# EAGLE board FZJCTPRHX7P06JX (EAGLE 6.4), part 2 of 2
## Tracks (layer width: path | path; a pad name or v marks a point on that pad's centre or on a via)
CLOCK  (via drill 0.6 pad 1.27)
  Top 0.406: v26.16,28.7 26.16,24.64 27.69,23.11 29.46,23.11 38.1,14.48 40.64,14.48 41.27,13.84 IC1.11 | IC21.4 30.25,6.58 29.46,7.37 29.46,17.27 22.86,23.88 v22.86,28.7 22.86,32.51 12.19,43.18 v12.19,50.04 13.46,51.31 15.75,51.31 16.33,50.72 IC3.11 | IC2.11 28.27,32.44 27.43,33.27 v26.16,33.27 | IC4.11 16.33,69.52 14.99,70.87 13.46,70.87 v11.94,69.34 11.94,56.9 v12.19,56.64 | IC6.11 39.8,81.86 v39.62,81.79 40.39,81.79 49.78,72.39 v54.1,72.39 | IC15.11 43.26,89.84 42.93,90.17 40.39,90.17 39.62,89.41 v39.62,86.87 | IC5.11 6.02,89.84 6.86,90.68 6.86,92.71 10.16,96.01 11.94,96.01 | v39.62,92.96 33.27,92.96 29.72,96.52 17.78,96.52 17.27,96.01 11.94,96.01 | IC10.11 73.84,8.71 72.39,10.16 v72.39,13.21 | IC7.11 54.03,63.32 v54.1,63.25 | v54.1,67.31 54.1,68.58 55.12,69.6 56.39,69.6 56.72,69.27 IC14.11 | v54.1,49.28 54.1,50.04 54.86,50.8 56.39,50.8 56.72,50.47 IC13.11 | IC9.11 65.96,25.73 v66.04,25.65 | v66.04,30.23 66.04,31.24 67.31,32.51 69.34,32.51 69.67,32.18 IC12.11 73.84,32.18 75.18,33.53 75.18,35.81 78.49,39.12 88.9,39.12 89.92,38.1 94.23,38.1 95,38.86 95,43.76 | IC8.11 v54.03,45.29 | v54.1,41.15 60.45,34.8 v66.04,34.8 | IC16.11 81.1,82.88 82.55,84.33 85.6,84.33 86.69,83.24 IC17.11 86.69,79.17 94.49,71.37 95,71.37 96.52,69.85 96.52,62.48 96.14,62.1 | IC18.11 93.9,62.05 94.23,61.72 95.76,61.72 96.14,62.1 | IC19.11 95,43.76 | 95,43.76 95.07,43.76 97.28,45.97 97.28,60.96 96.14,62.1 | v11.94,95.25 11.94,96.01 | IC11.11 80.09,14.4 v79.5,14.99
  Bottom 0.406: v26.16,33.27 v26.16,28.7 v22.86,28.7 | v12.19,56.64 v12.19,50.04 | v39.62,81.79 v39.62,86.87 v39.62,92.96 | v54.1,72.39 v54.1,67.31 v54.1,63.25 v54.1,49.28 54.03,49.2 v54.03,45.29 54.03,41.22 v54.1,41.15 | v66.04,34.8 v66.04,30.23 v66.04,25.65 66.04,19.56 v72.39,13.21 74.17,14.99 v79.5,14.99 | v11.94,69.34 v11.94,95.25
CLOCK2  (via drill 0.6)  (2 unrouted)
  Top 0.305: IC20.17 180.34,8.89 179.2,10.03 IC22.11 179.2,15.11 v180.34,16.26 | v192.02,16.76 192.15,16.64 IC23.11 | IC24.11 181.23,33.4 v181.1,33.53
  Bottom 0.305: v180.34,16.26 v192.02,16.76
D8
  Top 0.406: U$1.11 7.37,5.84 11.68,1.52 20.57,1.52 21.34,2.29 21.34,4.06 22.58,5.31 IC21.18
D11
  Top 0.406: U$1.14 19.53,6.58 IC21.17
D13
  Top 0.406: U$1.16 20.32,10.92 21.34,9.91 21.34,8.89 22.38,7.85 IC21.16
DATA
  Top 0.406: IC21.3 35.28,5.31 40.01,10.03 IC1.14
DATA2  (1 unrouted)
  Top 0.305: IC20.15 183.67,11.4 183.01,12.06 IC22.14
GND  (via drill 0.6, 0.6 pad 1.27)  (3 unrouted)
  Top 0.305: v179.32,5.59 179.43,5.7 IC20.21 188.36,5.7 188.47,5.59 | 188.47,5.59 188.47,5.08 188.65,4.9 IC20.3 191.59,4.9 192.02,5.33 | 188.47,5.59 188.47,6.35 188.61,6.5 IC20.5 | IC24.13 185.55,30.86 186.94,32.26 186.94,35.31 187.58,35.94 IC24.8 190.63,35.94 191.52,35.05 193.29,35.05 194.69,33.66 U$52.- | IC23.13 194.69,17.02 193.93,17.78 189.99,17.78 189.61,18.16 IC23.8 | U$53.- 193.55,10.16 192.53,9.14 192.53,5.84 192.02,5.33 | U$75.1 S1.P$1 174.9,22.96 176.66,21.21 IC22.8 176.66,17.65 v177.04,17.27 | v181.61,17.27 181.74,17.14 IC22.13 181.74,12.06 v181.86,11.94 | U$63.1 192.26,5.1 192.02,5.33
  Top 0.406: 38.99,11.56 39.24,11.3 IC1.13 46.1,11.3 46.99,12.19 46.99,15.75 47.62,16.38 IC1.8 49.02,16.41 v49.02,18.03 | 38.99,11.56 36.35,14.2 | 36.35,14.2 28.96,21.59 27.18,21.59 24.64,24.13 24.64,29.46 25.15,29.97 | IC21.10 36.35,14.2 | 25.15,29.97 25.4,30.23 27.69,30.23 28.02,29.9 IC2.13 33.45,29.9 34.04,30.48 34.04,34.29 34.72,34.98 IC2.8 | IC3.8 22.78,53.26 22.1,52.58 22.1,49.02 21.26,48.18 IC3.13 15.67,48.18 v15.24,47.75 | IC5.8 8.56,92.38 7.87,91.69 7.87,88.14 7.04,87.3 IC5.13 1.6,87.3 v1.52,87.38 | IC15.8 49.2,92.38 48.51,91.69 48.51,88.14 47.68,87.3 IC15.13 42.85,87.3 39.95,84.4 IC6.13 35.13,84.4 33.53,82.8 33.53,80.01 32.84,79.32 IC6.8 30.48,79.32 | J1.2 6.6,73.91 v1.52,78.99 | v15.24,67.06 15.32,66.98 IC4.13 20.75,66.98 21.84,68.07 21.84,71.63 22.28,72.06 IC4.8 24.56,72.06 v25.15,72.64 | IC11.8 86.54,16.94 85.85,16.26 85.85,13.72 84,11.86 IC11.13 79.93,11.86 79.32,11.25 v78.23,11.25 | IC13.8 62.66,53.01 61.47,51.82 61.47,49.53 59.87,47.93 IC13.13 57.96,47.83 IC8.13 49.61,47.83 v49.02,47.24 48.77,46.99 48.77,44.2 47.32,42.75 IC8.8 | 47.07,60.78 48.26,61.98 48.26,64.77 49.35,65.86 IC7.13 54.69,65.86 55.55,66.73 IC14.13 59.87,66.73 61.47,68.33 61.47,70.87 62.41,71.81 IC14.8 64.11,73.05 v63.5,73.66 | 47.07,60.78 IC7.8 | IC18.13 90.75,64.59 89.15,62.99 89.15,60.2 88.47,59.51 88.39,59.51 | 88.39,59.51 IC18.8 | IC19.13 90.75,46.3 89.28,44.83 | 89.28,44.83 88.9,44.45 88.9,41.91 88.21,41.22 IC19.8 84.51,41.22 v84.33,41.4 v75.69,41.4 | 47.07,60.78 47.07,56.31 v49.02,54.36 | IC17.8 82.6,87.43 80.59,85.42 IC16.13 77.04,85.42 75.69,84.07 75.69,82.04 73.99,80.34 IC16.8 72.49,79.91 74.68,77.72
  Top 0.406: IC17.13 89.23,79.93 91.19,77.98 v91.69,77.98 | v80.01,77.98 79.76,77.72 74.68,77.72 | v71.37,77.47 71.63,77.72 74.68,77.72 | v79.25,36.32 78.28,35.36 IC12.8 | v56.13,21.59 57.56,23.01 IC9.8 59.26,23.19 60.71,24.64 60.71,26.92 62.05,28.27 IC9.13 66.37,28.27 67.74,29.64 IC12.13 75.62,29.64 v75.69,29.72 75.69,27.43 76.2,26.92 76.2,24.89 77.22,23.88 v77.47,23.88 | 30.3,79.32 30.48,79.32 | v25.15,75.69 26.85,75.69 30.48,79.32 | IC21.19 28.47,4.04 29.74,2.77 IC21.1 36.8,2.77 v37.59,3.56 | U$1.23 19.3,28.7 v21.34,30.73 | v24.38,30.73 25.15,29.97 | v89.15,45.47 89.28,44.83 | v89.15,55.63 88.39,56.39 88.39,59.51 | IC10.13 v78.23,11.25 | v77.72,16.76 78.23,16.26 v78.23,11.25 | v71.37,4.32 70.1,5.59 IC10.8 | v37.59,9.91 37.59,10.16 38.99,11.56 | U$53.- IC23.13
  Top 0.61: U$1.4 2.29,23.62 1.52,24.38 1.52,35.81 6.6,40.89 | J4.2 6.6,40.89 | C1.- 10.67,36.83 6.6,40.89
  Top 0.813: J4.2 v6.6,47.75 J3.2 J2.2 v6.6,67.06 J1.2 | U$1.4 7.62,23.62 12.7,28.7 U$1.23
  Bottom 0.305: v179.32,5.59 179.32,9.4 v181.86,11.94 | U$52.- U$53.- | v177.04,17.27 v181.61,17.27
  Bottom 0.406: v6.6,47.75 v15.24,47.75 | v1.52,78.99 v1.52,87.38 | v15.24,67.06 v6.6,67.06 | v49.02,54.36 v49.02,47.24 | v91.69,77.98 v80.01,77.98 | v63.5,73.66 67.31,77.47 v71.37,77.47 | v79.25,36.32 v84.33,41.4 | v49.02,18.03 52.58,21.59 v56.13,21.59 | v25.15,72.64 v25.15,75.69 | v21.34,30.73 v24.38,30.73 | v89.15,55.63 v89.15,45.47 | v75.69,29.72 v75.69,41.4 | v77.47,23.88 77.72,23.62 v77.72,16.76 | v78.23,11.25 71.37,4.39 v71.37,4.32 | v37.59,3.56 v37.59,9.91
  pour Top (isolate 0.61): 0.76,99.31 99.06,99.31 99.06,1.02 99.06,0.76 0.76,0.76
LATCH  (via drill 0.6 pad 1.27)  (2 unrouted)
  Top 0.406: IC2.12 27.76,31.17 27.43,31.5 25.65,31.5 13.72,43.43 13.72,49.02 v14.48,49.78 15.75,49.78 16.08,49.45 IC3.12 | IC4.12 16.08,68.25 15.75,68.58 14.73,68.58 v14.22,69.09 13.46,68.33 13.46,57.4 v14.48,56.39 | IC15.12 41.33,88.57 v41.15,88.39 | IC5.12 2.36,88.57 1.52,89.41 1.52,94.49 5.59,98.55 v14.22,98.55 33.53,98.55 37.34,94.74 v41.15,94.74 | IC7.12 55.7,64.59 v55.88,64.77 | v55.88,68.07 55.96,68 IC14.12 | IC10.12 74.6,9.98 73.91,10.67 v73.91,11.68 | v55.88,73.41 55.37,73.91 49.78,73.91 41.15,82.55 v41.15,83.31 40.97,83.13 IC6.12 | IC8.12 55.8,46.56 v55.88,46.48 | v55.88,49.28 57.99,49.28 IC13.12 | v68.33,30.99 68.4,30.91 IC12.12 74.35,30.91 76.2,32.77 76.2,35.31 78.99,38.1 88.39,38.1 90.68,35.81 v95.5,35.81 | IC9.12 67.39,27 v68.33,27.94 | v55.88,41.91 61.47,36.32 67.06,36.32 68.07,35.31 v68.33,35.31 | IC16.12 80.85,84.15 82.04,85.34 86.36,85.34 87.96,83.74 IC17.12 87.96,79.68 95,72.64 95.76,72.64 98.3,70.1 v98.3,63.25 | v94.74,63.25 94.67,63.32 IC18.12 | IC19.12 94.56,45.03 95.89,46.35 | 95.89,46.35 96.01,46.48 96.01,54.86 v94.74,56.13 | v95.5,46.74 95.89,46.35 | IC1.12 40.01,12.57 v39.88,12.7 | IC11.12 79.58,13.13 v79.5,13.21 | IC21.2 36.04,4.04 37.34,5.33 38.61,5.33 v39.88,6.6
  Bottom 0.406: v14.48,56.39 v14.48,49.78 | v41.15,83.31 v41.15,88.39 v41.15,94.74 | v55.88,73.41 v55.88,68.07 v55.88,64.77 v55.88,49.28 v55.88,46.48 v55.88,41.91 | v68.33,27.94 v68.33,30.99 v68.33,35.31 | v98.3,63.25 v94.74,63.25 v94.74,56.13 | v95.5,35.81 v95.5,46.74 | v14.22,69.09 v14.22,98.55 | v39.88,12.7 v39.88,6.6 | v73.91,11.68 75.44,13.21 v79.5,13.21
LATCH2  (via drill 0.6)  (1 unrouted)
  Top 0.254: 180.47,11.3 183.13,8.64
  Top 0.305: IC23.12 193.42,12.32 192.79,11.68 184.91,11.68 184.47,11.25 IC20.14 184.47,8.96 184.15,8.64 183.13,8.64 | IC22.12 180.47,11.3 | IC24.12 181.23,32.13 v181.1,32
MISO  (1 unrouted)
N$1  (1 unrouted)
  Top 0.61: U$1.5 2.29,21.08
  Top 0.813: R160.1 113.26,99.97 U$55.1
N$2
  Top 0.61: 100.08,10.16 161.04,10.16 | 100.08,20.32 161.04,20.32 | 100.08,30.48 161.04,30.48 | 100.08,40.64 161.04,40.64 | 100.08,50.8 161.04,50.8 | 100.08,60.96 161.04,60.96 | 100.08,71.12 161.04,71.12 | 100.08,81.28 161.04,81.28 | 100.08,0 110.24,0 | 110.24,0 120.4,0 | 120.4,0 130.56,0 | 130.56,0 140.72,0 | 140.72,0 150.88,0 | 100.08,91.44 110.24,91.44 | 110.24,91.44 120.4,91.44 | 120.4,91.44 130.56,91.44 | 130.56,91.44 140.72,91.44 | 140.72,91.44 150.88,91.44 | 150.88,91.44 161.04,91.44 161.04,81.28 | 110.24,0 110.24,91.44 | 120.4,0 120.4,91.44 | 130.56,0 130.56,91.44 | 140.72,0 140.72,91.44 | 150.88,0 150.88,91.44 | 161.04,10.16 161.04,0 150.88,0 | 161.04,10.16 161.04,20.32 | 161.04,20.32 161.04,30.48 | 161.04,30.48 161.04,40.64 | 161.04,40.64 161.04,50.8 | 161.04,50.8 161.04,60.96 | 161.04,60.96 161.04,71.12 | 161.04,71.12 161.04,81.28 | 100.08,91.44 100.08,100.08 0,100.08 0,0 100.08,0 | 100.08,91.44 100.08,0
N$3  (via drill 0.6 pad 1.78)
  other vias: 2.29,21.08
N$4
  Top 0.305: IC22.15 184.28,14.86 185.74,16.32 R168.1
N$5
  Top 0.406: R81.2 74.67,2.75 U$28.1
N$6  (via drill 0.6 pad 1.27)
  Top 0.406: IC10.9 78.92,6.17 v79.25,5.84 | v79.25,9.14 79.25,9.65 80.19,10.59 IC11.14
  Bottom 0.406: v79.25,5.84 v79.25,9.14
N$7
  Top 0.305: IC22.1 187.71,21.74 R151.1
N$8
  Top 0.305: IC22.2 184.28,21.53 R152.1
N$9
  Top 0.305: R168.2 U$54.1
N$10
  Top 0.305: R151.2 U$56.1
N$11
  Top 0.305: R152.2 U$57.1
N$12
  Top 0.305: R169.2 U$58.1
N$13
  Top 0.305: R153.2 U$59.1
N$14
  Top 0.305: R154.2 U$60.1
N$15
  Top 0.305: U$61.1 173.04,12.89 R170.2
N$16
  Top 0.305: U$62.1 173.04,20.64 R155.2
N$17
  Top 0.305: IC22.3 183.01,22.29 R169.1
N$18
  Top 0.305: IC22.4 181.74,20.95 180.85,21.84 180.85,22.67 R153.1
N$19
  Top 0.305: IC22.5 180.47,20.95 179.83,21.59 179.14,21.59 R154.1
N$20
  Top 0.305: R170.1 175.45,15.24 178.05,15.24 179.2,16.38 IC22.6
N$21
  Top 0.305: IC22.7 177.93,18.67 178.31,18.29 178.31,16.76 177.55,16 176.28,16 174.94,17.34 R155.1
N$22
  Top 0.305: IC23.15 197.23,11.81 197.87,11.18 198.82,11.18 R156.1
N$23  (1 unrouted)
N$24
  Top 0.305: R171.2 202.95,18.1 U$66.1
N$25
  Top 0.305: R157.2 202.44,15.17 U$67.1
N$26
  Top 0.305: R158.2 202.69,21.66 U$68.1
N$27  (1 unrouted)
N$28  (1 unrouted)
N$29
  Top 0.406: IC1.15 45.59,8.76 46.99,7.37 46.99,6.1 50.77,2.31 R1.1
N$30
  Top 0.406: IC1.1 51.97,4.57 R2.1
N$31
  Top 0.406: IC1.2 50.67,8.76 52.6,6.83 R3.1
N$32
  Top 0.406: R1.2 58.41,2.31 U$2.3
N$33
  Top 0.406: R2.2 U$2.2
N$34
  Top 0.406: R3.2 58.41,6.83 U$2.1
N$35
  Top 0.406: R4.2 58.36,9.12 U$3.3
N$36
  Top 0.406: R5.2 58.6,11.35 U$3.2
N$37
  Top 0.406: R6.2 58.52,13.59 U$3.1
N$38
  Top 0.406: R7.2 58.31,15.93 U$4.3
N$39
  Top 0.406: R8.2 58.6,18.36 U$4.2
N$40
  Top 0.406: IC1.3 52.44,10.03 R4.1
N$41
  Top 0.406: IC1.4 54.27,11.3 R5.1
N$42
  Top 0.406: IC1.5 51.94,12.57 52.96,13.59 R6.1
N$43
  Top 0.406: IC1.6 51.27,13.84 R7.1
N$44
  Top 0.406: IC1.7 50.67,15.11 51.56,16 51.56,17.53 52.4,18.36 R8.1
N$45
  Top 0.406: R9.1 37.31,20.6 34.04,23.88 34.04,26.16 32.84,27.36 IC2.15
N$46
  Top 0.406: R9.2 43.8,20.07 58.45,20.07 U$4.1
N$47
  Top 0.406: R10.2 45.08,22.99 U$5.3
N$48
  Top 0.406: R11.2 45.47,25.38 U$5.2
N$49
  Top 0.406: R12.2 45.43,27.61 U$5.1
N$50
  Top 0.406: R13.2 45.26,29.79 U$6.3
N$51
  Top 0.406: R14.2 45.49,32.13 U$6.2
N$52
  Top 0.406: R15.2 45.26,34.37 U$6.1
N$53
  Top 0.406: R16.2 34.73,37.31 U$7.3
N$54
  Top 0.406: R17.2 33.78,39.14 U$7.2
N$55
  Top 0.406: R18.2 34.02,41.38 U$7.1
N$56
  Top 0.406: R19.2 33.17,43.66 U$8.3
N$57
  Top 0.406: R20.2 33.2,45.9 U$8.2
N$58
  Top 0.406: R21.2 32.96,48.13 U$8.1
N$59
  Top 0.406: R22.2 32.84,50.47 U$9.3
N$60
  Top 0.406: R23.2 U$9.2
N$61
  Top 0.406: R24.2 33.04,55.14 U$9.1
N$62
  Top 0.406: R25.2 33.01,57.53 U$10.3
N$63
  Top 0.406: R26.2 33.1,59.92 U$10.2
N$64
  Top 0.406: R27.2 32.86,62.15 U$10.1
N$65
  Top 0.406: R28.2 32.94,64.59 U$11.3
N$66
  Top 0.406: R29.2 33.17,66.93 U$11.2
N$67
  Top 0.406: R30.2 32.94,69.16 U$11.1
N$68
  Top 0.406: U$12.3 33.28,71.4 R31.2
N$69
  Top 0.406: U$12.2 32.99,73.69 R32.2
N$70  (via drill 0.6 pad 1.27)
  Top 0.406: R33.2 18.35,76.96 v21.84,76.96 | v33.53,76.96 33.53,75.15 U$12.1
  Bottom 0.406: v21.84,76.96 v33.53,76.96
N$71
  Top 0.406: R34.2 19.07,80.49 U$13.3
N$72
  Top 0.406: R35.2 19.1,82.73 U$13.2
N$73
  Top 0.406: R36.2 18.87,84.96 U$13.1
N$74
  Top 0.406: R37.2 18.99,87.3 U$14.3
N$75
  Top 0.406: R38.2 U$14.2
N$76
  Top 0.406: R39.2 19.2,91.97 U$14.1
N$77
  Top 0.406: U$15.3 16.67,94.89 R40.2
N$78
  Top 0.406: R41.2 22.61,93.5 U$15.2
N$79
  Top 0.406: R42.2 22.37,91.26 U$15.1
N$80
  Top 0.406: R43.2 22.31,89.08 U$16.3
N$81
  Top 0.406: R44.2 22.07,86.74 U$16.2
N$82
  Top 0.406: R45.2 22.31,84.51 U$16.1
N$83
  Top 0.406: U$17.3 22.73,82.27 R46.2
N$84
  Top 0.406: R47.2 23.08,80.95 U$17.2
N$85
  Top 0.406: U$17.1 23.25,77.75 R48.2
N$86
  Top 0.406: R49.2 36.18,74.95 U$18.3
N$87
  Top 0.406: R50.2 36.14,72.72 U$18.2
N$88
  Top 0.406: R51.2 36.38,70.48 U$18.1
N$89
  Top 0.406: R52.2 36.25,68.15 U$19.3
N$90
  Top 0.406: R53.2 U$19.2
N$91
  Top 0.406: R54.2 36.3,63.73 U$19.1
N$92
  Top 0.406: R55.2 36.58,61.59 U$20.3
N$93
  Top 0.406: R56.2 36.2,59.21 U$20.2
N$94
  Top 0.406: R57.2 36.48,56.72 U$20.1
N$95
  Top 0.406: R58.2 36.41,54.53 U$21.3
N$96
  Top 0.406: R59.2 36.17,52.2 U$21.2
N$97
  Top 0.406: R60.2 36.41,49.96 U$21.1
N$98
  Top 0.406: R61.2 36.48,47.73 U$22.3
N$99
  Top 0.406: R62.2 36.2,45.44 U$22.2
N$100
  Top 0.406: R63.2 36.33,43.2 U$22.1
N$101
  Top 0.406: R64.2 47.83,38.98 U$23.3
N$102
  Top 0.406: R65.2 48.26,37.41 U$23.2
N$103
  Top 0.406: R66.2 48.19,35.18 U$23.1
N$104
  Top 0.406: R67.2 48.32,32.84 U$24.3
N$105
  Top 0.406: R68.2 U$24.2
N$106
  Top 0.406: R69.2 48.37,28.42 U$24.1
N$107
  Top 0.406: R70.2 48.39,26.04 U$25.3
N$108
  Top 0.406: R71.2 48.26,23.9 U$25.2
N$109
  Top 0.406: R72.2 48.29,21.67 U$25.1
N$110
  Top 0.406: R73.2 61.42,20.5 U$26.3
N$111
  Top 0.406: R74.2 61.19,18.16 U$26.2
N$112
  Top 0.406: R75.2 61.42,15.93 U$26.1
N$113
  Top 0.406: R76.2 61.5,13.69 U$27.3
N$114
  Top 0.406: R77.2 61.21,11.4 U$27.2
N$115
  Top 0.406: R78.2 61.35,9.17 U$27.1
N$116
  Top 0.406: R79.2 61.32,6.88 U$28.3
N$117
  Top 0.406: R80.2 61.29,4.65 U$28.2
N$118
  Top 0.406: R82.2 97.1,5 U$29.3
N$119
  Top 0.406: R83.2 U$29.2
N$120
  Top 0.406: R84.2 97.05,9.42 U$29.1
N$121
  Top 0.406: R85.2 97.02,11.81 U$30.3
N$122
  Top 0.406: R86.2 97.1,14.2 U$30.2
N$123
  Top 0.406: R87.2 96.87,16.43 U$30.1
N$124
  Top 0.406: R88.2 90.05,20.71 88.75,19.41 U$31.3
N$125
  Top 0.406: R89.2 85.81,20.83 87.25,20.83 U$31.2
N$126
  Top 0.406: R90.2 87.1,22.68 U$31.1
N$127
  Top 0.406: R91.2 87.47,25.17 U$32.3
N$128
  Top 0.406: R92.2 87.76,27.46 U$32.2
N$129
  Top 0.406: R93.2 87.62,29.69 U$32.1
N$130
  Top 0.406: R94.2 87.65,31.98 U$33.3
N$131
  Top 0.406: R95.2 87.68,34.21 U$33.2
N$132
  Top 0.406: R96.2 87.45,36.45 U$33.1
N$133
  Top 0.406: R97.2 73.6,38.79 U$34.3
N$134
  Top 0.406: R98.2 U$34.2
N$135
  Top 0.406: R99.2 73.55,43.2 U$34.1
N$136
  Top 0.406: R100.2 73.27,45.59 U$35.3
N$137
  Top 0.406: R101.2 73.66,47.98 U$35.2
N$138
  Top 0.406: R102.2 73.63,50.22 U$35.1
N$139
  Top 0.406: R103.2 73.45,52.65 U$36.3
N$140
  Top 0.406: R104.2 73.69,54.99 U$36.2
N$141
  Top 0.406: R105.2 72.94,57.73 U$36.1
N$142
  Top 0.406: R106.2 73.37,59.97 U$37.3
N$143
  Top 0.406: R107.2 73.66,62.26 U$37.2
N$144
  Top 0.406: R108.2 73.53,64.49 U$37.1
N$145
  Top 0.406: R109.2 73.55,66.78 U$38.3
N$146
  Top 0.406: R110.2 73.58,69.01 U$38.2
N$147
  Top 0.406: R111.2 73.35,71.25 U$38.1
N$148
  Top 0.406: R112.2 65.22,75.18 61.07,75.18 U$39.3
N$149
  Top 0.406: R113.2 U$39.2
N$150
  Top 0.406: R114.2 59.96,80.29 U$39.1
N$151
  Top 0.406: R115.2 59.94,82.68 U$40.3
N$152
  Top 0.406: R116.2 60.02,85.06 U$40.2
N$153
  Top 0.406: R117.2 59.78,87.3 U$40.1
N$154
  Top 0.406: R118.2 59.86,89.74 U$41.3
N$155
  Top 0.406: R119.2 60.1,92.08 U$41.2
N$156
  Top 0.406: R120.2 59.86,94.31 U$41.1
N$157
  Top 0.406: R121.2 63.15,94.46 U$42.3
N$158
  Top 0.406: R122.2 62.87,92.18 U$42.2
N$159
  Top 0.406: R123.2 63,89.94 U$42.1
N$160
  Top 0.406: R124.2 62.97,87.66 U$43.3
N$161
  Top 0.406: R125.2 62.94,85.42 U$43.2
N$162
  Top 0.406: R126.2 63.18,83.19 U$43.1
N$163
  Top 0.406: R127.2 63.05,80.85 U$44.3
N$164
  Top 0.406: R128.2 U$44.2
N$165  (via drill 0.6 pad 1.27)
  Top 0.406: R129.2 94.17,76.71 96.01,76.71 v96.27,76.45 | 82.59,76.66 v82.8,76.45 82.55,76.71 74.68,76.71 73.91,75.95 69.85,75.95 69.13,76.66 U$44.1
  Bottom 0.406: v82.8,76.45 v96.27,76.45
N$166
  Top 0.406: R130.2 96.14,96.39 U$45.3
N$167
  Top 0.406: R131.2 93.75,96.77 U$45.2
N$168
  Top 0.406: R132.2 91.52,96.74 U$45.1
N$169
  Top 0.406: R133.2 89.33,96.56 U$46.3
N$170
  Top 0.406: R134.2 87,96.8 U$46.2
N$171
  Top 0.406: R135.2 84.76,96.56 U$46.1
N$172  (via drill 0.6 pad 1.27)
  Top 0.406: v81.28,96.77 82.53,95.53 R136.2
  Bottom 0.406: U$47.3 76.91,92.41 v76.96,92.46 v81.28,96.77
N$173
  Top 0.406: R137.2 77.47,73.64 U$47.2
N$174
  Top 0.406: R138.2 77.23,71.4 U$47.1
N$175
  Top 0.406: R139.2 77.07,69.11 U$48.3
N$176
  Top 0.406: R140.2 77.04,66.88 U$48.2
N$177
  Top 0.406: R141.2 77.27,64.64 U$48.1
N$178
  Top 0.406: R142.2 77.4,62.31 U$49.3
N$179
  Top 0.406: R143.2 U$49.2
N$180
  Top 0.406: R144.2 77.2,57.63 U$49.1
N$181
  Top 0.406: R145.2 77.48,54.48 U$50.3
N$182
  Top 0.406: R146.2 77.09,52.09 U$50.2
N$183
  Top 0.406: R147.2 77.12,49.86 U$50.1
N$184
  Top 0.406: R148.2 77.3,47.68 U$51.3
N$185
  Top 0.406: R149.2 77.11,45.49 U$51.2
N$186
  Top 0.406: R150.2 77.25,43.16 U$51.1
N$187  (1 unrouted)
N$188
  Top 0.305: R173.2 U$72.1
N$189
  Top 0.305: R162.2 U$73.1
N$190  (1 unrouted)
N$191
  Top 0.66: 24.89,14.22 27.18,14.22
N$192
  Top 0.66: 24.89,12.95 27.18,12.95
N$193
  Top 0.66: 24.64,11.68 27.18,11.68
N$194
  Top 0.66: 24.64,10.41 27.18,10.41
N$195
  Top 0.66: 24.89,9.14 27.18,9.14
N$196
  Top 0.406: R81.1 83.69,3.17 86.36,5.84 86.36,7.62 84.66,9.32 IC11.15
N$197
  Top 0.406: IC11.1 90.83,5 R82.1
N$198
  Top 0.406: IC11.2 89.74,9.32 91.87,7.19 R83.1
N$199
  Top 0.406: IC11.3 90.25,10.59 91.42,9.42 R84.1
N$200
  Top 0.406: IC11.4 91.91,11.86 R85.1
N$201
  Top 0.406: IC11.5 90.6,13.13 91.67,14.2 R86.1
N$202
  Top 0.406: IC11.6 90.09,14.4 92.13,16.43 R87.1
N$203
  Top 0.406: IC11.7 89.33,15.67 90.86,17.2 R88.1
N$204
  Top 0.406: IC12.15 73.99,27.1 74.68,26.42 74.68,24.64 77.47,21.84 80.26,21.84 81.66,20.45 R89.1
N$205
  Top 0.406: IC12.1 81.43,22.68 R90.1
N$206
  Top 0.406: IC12.2 80.64,27.1 R91.1
N$207
  Top 0.406: IC12.3 81.36,28.37 82.27,27.46 R92.1
N$208
  Top 0.406: IC12.4 83.48,29.64 R93.1
N$209
  Top 0.406: IC12.5 81.5,30.91 R94.1
N$210
  Top 0.406: IC12.6 79.93,32.18 81.97,34.21 R95.1
N$211
  Top 0.406: IC12.7 79.68,33.45 82.68,36.45 R96.1
N$212
  Top 0.406: IC13.15 61.04,45.39 61.98,44.45 61.98,41.91 65.1,38.79 R97.1
N$213
  Top 0.406: IC13.1 67.36,40.97 R98.1
N$214
  Top 0.406: IC13.2 65.86,45.39 68.05,43.2 R99.1
N$215
  Top 0.406: IC13.3 67.53,46.66 R100.1
N$216
  Top 0.406: IC13.4 69.51,47.93 R101.1
N$217
  Top 0.406: IC13.5 67.74,49.2 68.76,50.22 R102.1
N$218
  Top 0.406: IC13.6 66.41,50.47 R103.1
N$219
  Top 0.406: IC13.7 65.71,51.74 66.55,52.58 66.55,53.59 67.94,54.99 R104.1
N$220
  Top 0.406: IC14.15 60.27,64.19 61.98,62.48 61.98,60.96 65.2,57.73 R105.1
N$221
  Top 0.406: IC14.1 67.06,59.97 R106.1
N$222
  Top 0.406: IC14.2 66.37,64.19 68.3,62.26 R107.1
N$223
  Top 0.406: IC14.3 66.88,65.46 67.84,64.49 R108.1
N$224
  Top 0.406: IC14.4 68.54,66.73 R109.1
N$225
  Top 0.406: IC14.5 67.23,68 68.25,69.01 R110.1
N$226
  Top 0.406: IC14.6 66.73,69.27 68.71,71.25 R111.1
N$227
  Top 0.406: IC14.7 65.46,70.54 68.06,73.14 R112.1
N$228
  Top 0.406: IC15.15 47.57,84.76 48.51,83.82 48.51,81.79 52.25,78.05 R113.1
N$229
  Top 0.406: IC15.1 53.75,80.29 R114.1
N$230
  Top 0.406: IC15.2 52.4,84.76 54.48,82.68 R115.1
N$231
  Top 0.406: IC15.3 53.42,86.03 54.38,85.06 R116.1
N$232
  Top 0.406: IC15.4 R117.1
N$233
  Top 0.406: IC15.5 52.76,88.57 53.92,89.74 R118.1
N$234
  Top 0.406: IC15.6 52.25,89.84 54.48,92.08 R119.1
N$235
  Top 0.406: IC15.7 51.74,91.11 53.34,92.71 53.34,93.47 54.18,94.31 R120.1
N$236
  Top 0.406: IC16.15 75.87,87.96 74.68,89.15 74.68,89.66 73.91,90.42 73.91,92.46 71.91,94.46 R121.1
N$237
  Top 0.406: IC16.1 69.55,92.18 R122.1
N$238
  Top 0.406: IC16.2 70.79,87.96 68.81,89.94 R123.1
N$239
  Top 0.406: IC16.3 69.02,86.69 R124.1
N$240
  Top 0.406: IC16.4 R125.1
N$241
  Top 0.406: IC16.5 69.67,84.15 68.71,83.19 R126.1
N$242
  Top 0.406: IC16.6 70.43,82.88 68.4,80.85 R127.1
N$243
  Top 0.406: IC16.7 70.94,81.61 69.85,80.52 69.85,79.5 69.01,78.66 R128.1
N$244
  Top 0.406: IC17.15 91.77,79.93 92.93,78.78 R129.1
N$245
  Top 0.406: IC17.1 96.14,90.53 R130.1
N$246
  Top 0.406: IC17.2 91.77,89.23 93.75,91.21 R131.1
N$247
  Top 0.406: IC17.3 90.5,89.74 91.52,90.75 R132.1
N$248
  Top 0.406: IC17.4 89.23,91.61 R133.1
N$249
  Top 0.406: IC17.5 87.96,89.84 87,90.81 R134.1
N$250
  Top 0.406: IC17.6 86.69,89.59 84.76,91.52 R135.1
N$251
  Top 0.406: IC17.7 85.42,89.08 82.79,91.71 R136.1
N$252
  Top 0.406: IC18.15 90.86,67.13 88.65,69.34 88.65,71.37 86.39,73.64 R137.1
N$253
  Top 0.406: IC18.1 83.67,71.4 R138.1
N$254
  Top 0.406: IC18.2 84.26,67.13 R139.1
N$255
  Top 0.406: IC18.3 83.49,65.86 82.47,66.88 R140.1
N$256
  Top 0.406: IC18.4 81.37,64.59 R141.1
N$257
  Top 0.406: IC18.5 83.3,63.32 R142.1
N$258
  Top 0.406: IC18.6 84.91,62.05 82.73,59.87 R143.1
N$259
  Top 0.406: IC18.7 85.42,60.78 82.27,57.63 R144.1
N$260
  Top 0.406: IC19.15 90.86,48.84 88.65,51.05 88.65,52.58 86.74,54.48 R145.1
N$261
  Top 0.406: IC19.1 84.53,52.09 R146.1
N$262
  Top 0.406: IC19.2 84.51,48.84 83.49,49.86 R147.1
N$263
  Top 0.406: IC19.3 82.38,47.57 R148.1
N$264
  Top 0.406: IC19.4 84.4,46.3 83.57,45.47 81.29,45.47 R149.1
N$265
  Top 0.406: IC19.5 84.91,45.03 83.03,43.16 R150.1
N$266
  Top 0.66: 24.89,7.87 27.18,7.87
N$267
  Top 0.66: 24.89,6.6 27.18,6.6
N$268
  Top 0.66: 24.89,5.33 27.18,5.33
N$269
  Top 0.66: 24.89,4.06 27.18,4.06
N$270
  Top 0.66: 24.89,2.79 27.18,2.79
N$271
  Top 0.66: 34.04,14.22 31.5,14.22
N$272
  Top 0.66: 33.78,12.95 31.5,12.95
N$273
  Top 0.305: IC24.1 190.88,27.05 192.53,28.7 R163.1
N$274
  Top 0.305: R162.1 180.15,28.7 181.1,28.7 181.48,28.32 IC24.15
N$275
  Top 0.305: IC23.7 190.88,21.53 R173.1
N$276
  Top 0.406: IC10.7 68.66,7.44 68.07,6.86 68.07,5.33 67.39,4.65 R80.1
N$277
  Top 0.406: IC10.6 68.11,8.71 R79.1
N$278
  Top 0.406: IC10.5 67.13,9.98 66.32,9.17 R78.1
N$279
  Top 0.406: IC10.4 65.47,11.25 R77.1
N$280
  Top 0.406: IC10.3 67.45,12.52 R76.1
N$281
  Top 0.406: R75.1 66.88,15.93 69.01,13.79 IC10.2
N$282
  Top 0.406: IC10.1 67.26,18.16 R74.1
N$283
  Top 0.406: IC10.15 74.35,13.79 73.41,14.73 73.41,16 68.91,20.5 R73.1
N$284
  Top 0.406: IC9.7 56.21,24.46 55.12,23.37 55.12,22.86 53.92,21.67 R72.1
N$285
  Top 0.406: IC9.6 55.7,25.73 53.87,23.9 R71.1
N$286
  Top 0.406: IC9.5 54.29,27 R70.1
N$287
  Top 0.406: IC9.4 52.51,28.27 R69.1
N$288
  Top 0.406: IC9.3 54.79,29.54 53.67,30.66 R68.1
N$289
  Top 0.406: IC9.2 55.36,30.81 R67.1
N$290
  Top 0.406: IC9.1 54.46,35.18 R66.1
N$291
  Top 0.406: IC9.15 61.65,30.81 60.71,31.75 60.71,32.77 56.06,37.41 R65.1
N$292
  Top 0.406: IC8.7 44.27,44.02 42.93,42.67 42.93,40.9 R64.1
N$293
  Top 0.406: IC8.6 43.51,45.29 41.43,43.2 R63.1
N$294
  Top 0.406: IC8.5 43,46.56 41.88,45.44 R62.1
N$295
  Top 0.406: IC8.4 41.23,47.83 R61.1
N$296
  Top 0.406: IC8.3 42.85,49.1 41.99,49.96 R60.1
N$297
  Top 0.406: IC8.2 43.61,50.37 41.78,52.2 R59.1
N$298
  Top 0.406: IC8.1 42.62,54.53 R58.1
N$299
  Top 0.406: IC8.15 49.45,50.37 48.51,51.31 48.51,52.58 44.37,56.72 R57.1
N$300
  Top 0.406: IC7.7 43.76,62.05 42.93,61.21 42.93,60.2 41.94,59.21 R56.1
N$301
  Top 0.406: IC7.6 43.26,63.32 41.53,61.59 R55.1
N$302
  Top 0.406: IC7.5 42.75,64.59 41.88,63.73 R54.1
N$303
  Top 0.406: IC7.4 40.27,65.86 R53.1
N$304
  Top 0.406: IC7.3 42.15,67.13 R52.1
N$305
  Top 0.406: IC7.2 43.87,68.4 41.78,70.48 R51.1
N$306
  Top 0.406: IC7.1 42.37,72.72 R50.1
N$307
  Top 0.406: R49.1 43.66,74.95 47.5,71.12 47.5,69.6 48.26,68.83 49.53,68.83 49.96,68.4 IC7.15
N$308
  Top 0.406: IC6.7 30.05,80.59 27.2,77.75 R48.1
N$309
  Top 0.406: IC6.6 29.54,81.86 27.66,79.98 R47.1
N$310
  Top 0.406: IC6.5 27.77,83.13 R46.1
N$311
  Top 0.406: IC6.4 26.3,84.4 R45.1
N$312
  Top 0.406: IC6.3 28.37,85.67 27.3,86.74 R44.1
N$313
  Top 0.406: IC6.2 29.3,86.94 R43.1
N$314
  Top 0.406: R42.1 28.55,91.26 31.09,88.72 IC6.1
N$315
  Top 0.406: IC6.15 35.48,86.94 34.8,87.63 34.8,88.65 29.95,93.5 R41.1
N$316
  Top 0.406: IC5.7 11.35,91.11 14.24,94 R40.1
N$317
  Top 0.406: IC5.6 11.86,89.84 13.99,91.97 R39.1
N$318
  Top 0.406: IC5.5 12.37,88.57 13.54,89.74 R38.1
N$319
  Top 0.406: IC5.4 R37.1
N$320
  Top 0.406: IC5.3 12.52,86.03 13.59,84.96 R36.1
N$321
  Top 0.406: IC5.2 12.01,84.76 14.05,82.73 R35.1
N$322
  Top 0.406: IC5.1 12.9,80.49 R34.1
N$323
  Top 0.406: IC5.15 6.93,84.76 7.87,83.82 7.87,82.55 12.22,78.21 R33.1
N$324
  Top 0.406: IC4.7 25.58,70.79 28.47,73.69 R32.1
N$325
  Top 0.406: IC4.6 26.33,69.52 28.21,71.4 R31.1
N$326
  Top 0.406: IC4.5 26.85,68.25 27.76,69.16 R30.1
N$327
  Top 0.406: IC4.4 24.03,66.93 R29.1
N$328
  Top 0.406: IC4.3 27.09,65.71 R28.1
N$329
  Top 0.406: IC4.2 25.22,64.44 27.51,62.15 R27.1
N$330
  Top 0.406: IC4.1 27.23,59.92 R26.1
N$331
  Top 0.406: IC4.15 20.65,64.44 21.84,63.25 21.84,61.21 25.53,57.53 R25.1
N$332
  Top 0.406: IC3.7 25.32,51.99 26.42,53.09 26.42,54.36 27.2,55.14 R24.1
N$333
  Top 0.406: IC3.6 25.58,50.72 27.76,52.91 R23.1
N$334
  Top 0.406: IC3.5 27.19,49.45 R22.1
N$335
  Top 0.406: IC3.4 29.12,48.18 R21.1
N$336
  Top 0.406: IC3.3 26.49,46.91 27.51,45.9 R20.1
N$337
  Top 0.406: IC3.2 25.73,45.64 27.71,43.66 R19.1
N$338
  Top 0.406: IC3.1 27.08,41.38 R18.1
N$339
  Top 0.406: IC3.15 20.9,45.64 22.1,44.45 22.1,42.16 25.12,39.14 R17.1
N$340
  Top 0.406: IC2.7 37.52,33.71 38.35,34.54 38.35,37.3 R16.1
N$341
  Top 0.406: IC2.6 38.02,32.44 39.95,34.37 R15.1
N$342
  Top 0.406: IC2.5 38.53,31.17 39.5,32.13 R14.1
N$343
  Top 0.406: IC2.4 40.3,29.9 R13.1
N$344
  Top 0.406: IC2.3 38.43,28.63 39.45,27.61 R12.1
N$345
  Top 0.406: IC2.2 37.92,27.36 39.9,25.38 R11.1
N$346
  Top 0.406: IC2.1 39.22,22.99 R10.1
N$347
  Top 0.406: IC2.9 24.21,34.98 15.75,43.43 15.75,46.23 16.43,46.91 IC3.14
N$348
  Top 0.406: IC2.14 29.9,28.7 28.19,28.7 27.43,27.94 27.43,25.4 28.19,24.64 29.72,24.64 37.97,16.38 IC1.9
N$349
  Top 0.406: IC4.14 16.18,65.71 15.49,65.02 15.49,62.48 17.93,60.05 IC3.9
N$350
  Top 0.406: IC5.14 2.21,86.03 1.52,85.34 1.52,82.8 4.57,79.76 8.64,79.76 16.33,72.06 IC4.9
N$351  (via drill 0.6 pad 1.27)
  Top 0.406: IC5.9 3.76,94.44 6.35,97.03 15.75,97.03 16.26,97.54 31.75,97.54 v34.04,95.25 | v34.04,85.6 34.11,85.67 IC6.14
  Bottom 0.406: v34.04,95.25 v34.04,85.6
N$352  (via drill 0.6 pad 1.27)
  Top 0.406: IC6.9 39.34,77.22 43.43,77.22 49.02,71.63 v49.02,70.87 | v49.02,67.31 49.2,67.13 IC7.14
  Bottom 0.406: v49.02,70.87 v49.02,67.31
N$353  (1 unrouted)
N$354  (1 unrouted)
N$355  (1 unrouted)
N$356  (via drill 0.6 pad 1.27)
  Top 0.406: IC12.14 70.54,28.37 69.85,27.69 69.85,26.42 v69.34,25.91 | IC11.9 81.36,16.94 78.74,19.56 72.64,19.56 v69.34,22.86
  Bottom 0.406: v69.34,25.91 v69.34,22.86
N$357  (1 unrouted)
N$358  (1 unrouted)
N$359
  Top 0.406: IC15.14 43.1,86.03 42.67,85.6 42.67,82.55 50.29,74.93 56.39,74.93 57.96,73.36 IC14.9
N$360
  Top 0.406: IC15.9 44.4,94.44 47.75,97.79 73.66,97.79 80.77,90.68 80.77,87.38 80.09,86.69 IC16.14
N$361  (1 unrouted)
N$362
  Top 0.406: IC17.9 84.15,79.68 93.73,70.1 94.49,70.1 95.25,69.34 95.25,66.55 94.56,65.86 IC18.14
N$363
  Top 0.406: IC18.9 92.81,52.98 94.74,51.05 94.74,48.51 93.8,47.57 IC19.14
N$364
  Top 0.305: IC23.6 192.15,21.78 R161.1
N$365
  Top 0.305: IC23.5 193.42,20.7 197.87,25.15 R159.1
N$366
  Top 0.305: IC23.4 194.69,20.7 197.87,23.88 199.58,23.88 R172.1
N$367
  Top 0.305: IC23.3 195.96,20.7 196.85,21.59 R158.1
N$368
  Top 0.305: IC23.2 197.23,17.4 199.39,15.24 R157.1
N$369
  Top 0.305: IC23.1 200.47,17.61 R171.1
N$370  (via drill 0.6)  (1 unrouted)
  Top 0.305: IC23.9 189.21,13.44 v188.72,12.95 | IC24.14 181.48,29.59 v181.1,29.97
N$371  (1 unrouted)
N$372
  Top 0.66: 33.53,11.68 31.5,11.68
N$373
  Top 0.66: 33.78,10.41 31.5,10.41
N$374
  Top 0.305: U$75.2 171.91,25.69 U$64.1
N$375
  Top 0.305: U$64.2 174.5,27.69 U$52.+
  Bottom 0.305: U$53.+ U$52.+
N$376
  Top 0.66: 33.78,9.14 31.5,9.14
N$377
  Top 0.66: 33.78,7.87 31.5,7.87
N$378
  Top 0.66: 33.78,6.6 31.5,6.6
N$379
  Top 0.66: 33.78,5.33 31.5,5.33
N$380
  Top 0.66: 33.78,4.06 31.5,4.06
N$381
  Top 0.66: 34.04,2.79 31.5,2.79
RESET2
  Top 0.305: S1.P$2 170.43,10.16 175.6,4.99 R176.1 179.74,2.03 180.59,2.03 182.37,0.25 186.18,0.25 | U$63.3 193.02,2.03 191.01,2.03 189.23,0.25 186.18,0.25 | IC20.29 186.07,0.36 186.18,0.25
VCC  (via drill 0.6, 0.6 pad 1.27)  (3 unrouted)
  Top 0.305: IC22.10 177.93,9.78 178.94,8.76 | 178.94,8.76 179.58,8.13 181.35,8.13 IC20.18 182.4,8.1 183.2,7.3 IC20.6 191.33,7.3 | 191.33,7.3 191.52,7.11 191.52,6.1 191.12,5.7 IC20.4 | IC24.10 185.55,34.67 v185.67,34.54 | v185.67,28.7 185.67,27.69 185.04,27.05 IC24.16 181.48,27.05 180.85,27.69 178.31,27.69 176.31,29.69 U$64.3 | IC23.16 198.5,14.86 197.87,15.49 v196.6,15.49 | R176.2 178.85,8.76 178.94,8.76 | 191.33,7.3 191.52,7.48 191.52,9.91 v191.01,10.41 | IC23.10 190.88,15.37 v191.01,15.49 189.48,15.49 187.43,13.44 IC22.16
  Top 0.406: IC1.16 44.58,7.49 45.47,6.6 v45.47,5.84 45.47,2.79 44.2,1.52 25.55,1.52 IC21.20 | IC2.16 31.83,26.09 32.51,25.4 v32.51,24.38 32.51,23.62 38.35,17.78 v45.47,17.78 45.47,16 44.58,15.11 IC1.10 | IC3.16 19.63,44.37 20.57,43.43 v20.57,42.67 20.57,41.91 25.65,36.83 32.26,36.83 v32.51,36.58 32.51,34.29 31.93,33.71 IC2.10 | IC4.16 19.38,63.17 20.32,62.23 v20.32,61.47 20.32,55.12 v20.57,54.86 20.57,52.83 19.74,51.99 IC3.10 16.59,51.99 16,52.58 J3.1 | IC5.16 5.66,83.49 6.35,82.8 v6.35,82.04 | IC15.16 46.05,83.49 46.99,82.55 v46.99,82.04 46.99,80.52 v48.26,79.25 51.31,76.2 56.9,76.2 59.44,73.66 v60.45,73.66 60.45,71.37 59.61,70.54 IC14.10 56.72,70.54 56.39,70.87 52.76,70.87 IC7.16 | J1.1 9.14,74.42 v6.35,77.22 | IC4.10 19.48,70.79 19.81,71.12 19.81,73.66 v20.32,74.17 27.18,74.17 31.24,78.23 33.53,78.23 35.89,80.59 IC6.10 38.53,80.59 v39.88,79.25 | U$1.21 20.32,23.62 v21.08,24.38 | v46.99,93.98 46.99,92.05 46.05,91.11 IC15.10 44.32,91.19 39.12,91.19 37.24,89.31 IC6.16 | IC5.10 5.26,91.11 5.84,91.69 5.84,94.23 v6.35,94.74 | IC7.10 49.86,62.05 49.28,61.47 49.28,57.4 51.56,55.12 51.56,51.74 IC8.16 52.09,52.07 56.64,52.07 56.9,51.82 57.99,51.82 IC13.10 59.61,51.74 60.45,52.58 v60.45,55.12 v60.45,60.71 60.45,61.98 59.51,62.92 IC14.16 | 82.88,8.05 IC11.16 82.3,7.9 82.3,6.35 | IC10.10 79.93,7.44 81.03,6.35 82.3,6.35 | 82.3,6.35 v84.58,6.35 | v74.17,36.83 74.17,34.04 73.58,33.45 IC12.10 70.43,33.45 70.1,33.78 66.8,33.78 65.1,32.08 IC9.16 | 72.47,25.83 IC12.16 70.76,24.46 | IC18.10 91.01,60.78 90.17,59.94 v90.17,57.66 90.68,57.15 v90.68,51.82 90.68,50.8 91.36,50.11 IC19.16
  Top 0.406: IC18.16 91.62,68.4 v90.17,69.85 90.17,71.88 82.8,79.25 v75.44,79.25 75.44,80.01 77.04,81.61 IC16.10 81.61,81.61 83.31,83.31 85.09,83.31 85.42,82.98 IC17.10 | IC19.10 91.01,42.49 90.68,42.16 v90.68,40.13 77.47,40.13 v74.17,36.83 | IC8.10 53.01,44.02 53.59,43.43 57.38,43.43 IC13.16 59.77,44.12 60.45,43.43 v60.45,42.16 60.45,41.15 64.01,37.59 67.82,37.59 68.58,36.83 v74.17,36.83 | IC17.16 95.5,81.28 98.04,78.74 98.04,76.2 96.52,74.68 v95,74.68 | IC9.10 70.76,24.46 | 70.76,24.46 72.11,23.11 v74.17,23.11 76.71,20.57 79.76,20.57 82.04,18.29 v84.58,18.29 84.58,16.26 84,15.67 IC11.10 80.85,15.67 78.23,18.29 76.96,18.29 76.25,17.58 IC10.16 | v75.44,90.93 77.14,89.23 IC16.16
  Top 0.61: J4.1 9.14,42.93 C1.+
  Top 0.813: J1.1 J2.1 J3.1 J4.1
  Bottom 0.305: v185.67,34.54 v185.67,28.7 | v196.6,15.49 v191.01,15.49 v191.01,10.41 194.09,7.33 U$63.2
  Bottom 0.406: v32.51,36.58 v32.51,24.38 v21.08,24.38 | v20.57,54.86 v20.57,42.67 | v6.35,77.22 v6.35,82.04 v6.35,94.74 | v20.32,74.17 v20.32,61.47 | v45.47,5.84 v45.47,17.78 | v46.99,82.04 v46.99,93.98 | v39.88,79.25 v48.26,79.25 | v84.58,18.29 v84.58,6.35 | v74.17,36.83 v74.17,23.11 | v60.45,55.12 v60.45,42.16 | v60.45,73.66 v60.45,60.71 | v75.44,79.25 v75.44,90.93 | v90.17,57.66 v90.17,69.85 v95,74.68 | v90.68,40.13 v90.68,51.82
(copper drawn outside any net)
  shapes: Top circle x1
